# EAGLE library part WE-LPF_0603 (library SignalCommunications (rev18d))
Multilayer Chip Low-Pass Filter Characteristics Operating temperature: –40 °C to +85 °C Power capacity up to 3 W Low insertion loss and high attenuation in the stop-band Applications RF applications Wireless communication systems like DECT, PACS, PHS, GSM, WLAN, Bluetooth … Details see: http://katalog.we-online.de/en/pbs/WE-LPF? Updated by Dan Xu 2014-07-08 2014 (C) Wurth Elektronik
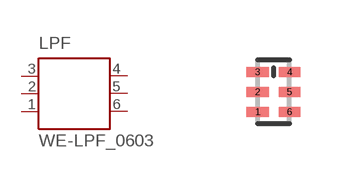
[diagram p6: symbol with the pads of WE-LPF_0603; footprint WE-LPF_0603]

Designator prefix LPF

## WE-LPF_0603_748112024  [WE-LPF_0603]
1  1  pas
2  2  pas
3  3  pas
4  4  pas
5  5  pas
6  6  pas

## Footprint WE-LPF_0603 (pad centres in mm)
Multilayer Chip Low-Pass Filters WE-LPF
smd 0.55 x 0.25: 1 -0.4,-0.5; 2 -0.4,0; 3 -0.4,0.5; 4 0.4,0.5; 5 0.4,0; 6 0.4,-0.5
